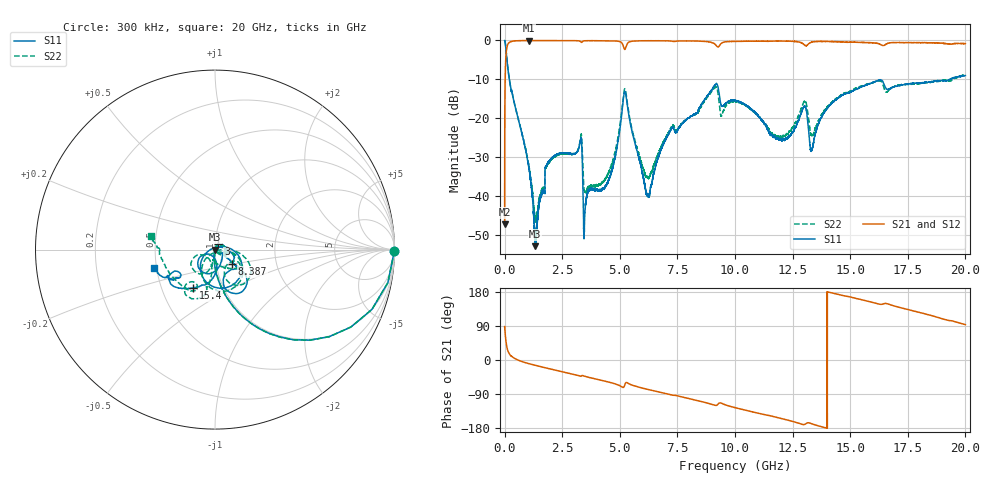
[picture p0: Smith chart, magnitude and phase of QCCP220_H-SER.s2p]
!{QCCP220}
!Johanson Technology Inc.
!www.johansontechnology.com
!Test Board Conditions:
!Substrate Type  RO4350B
!Substrate Thickness  20 mil
!Substrate Dk  3.66
!TL Type: GCPW
!TL Trace Width  36 mil
!TL Gap  12 mil
!Electrode orientation  Horizontal
!DUT TOPOLOGY	SERIES
!Mounting Pad LxW  26x36 mil
! Created Sat Jan  9 18:34:06 2021
# hz S ma R 50
! 2 Port Network Data from SP1.SP block
! freq  magS11  angS11  magS21  angS21  magS12  angS12  magS22  angS22
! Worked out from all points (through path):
!   20001 points, 300 kHz to 20 GHz, reference 50 ohm
!   highest |S21| = -0.02 dB at 1.049 GHz (marker M1); lowest = -47.3 dB at 300 kHz (marker M2)
!   group delay of S21, straight-line fit = 37.2 ps
!   lowest |S11| = -52.9 dB at 1.332 GHz (marker M3), VSWR 1.00, Z = 49.8 - j0.0174 ohm
!   |S11| at or under -10 dB: 205.2 MHz to 19.33 GHz (19.13 GHz wide, 196 % of centre)
!   |S22| runs from -46.7 to 0.0 dB; largest |S21 - S12| = 0.017
!   S11 on the Smith chart (normalised r, x): 300 kHz: open; 3 GHz: 1.04, +0.06; 8.387 GHz: 1.20, -0.19; 15.4 GHz: 0.72, -0.33; 20 GHz: 0.48, -0.11
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300000  0.9987 -0.5  0.0043 88.1  0.004282 89.0  1 -0.5
1.433e8  0.4341 -65.5  0.897 24.3  0.8978 24.2  0.4364 -65.4
1.0493e9  0.0236 -103.0  0.9981 -9.5  0.9976 -9.5  0.0249 -91.0
1.3323e9  0.002264 -175.6  0.9957 -14.1  0.9969 -14.0  0.005051 -31.8
1.8503e9  0.02568 65.8  0.9964 -21.7  0.9957 -21.7  0.02498 71.1
3.0003e9  0.03501 57.8  0.9935 -37.7  0.9938 -37.7  0.03477 46.3
3.3343e9  0.05381 -7.8  0.9443 -42.2  0.9445 -42.2  0.06104 -14.7
3.5003e9  0.0074 63.4  0.9906 -43.3  0.9903 -43.4  0.01128 -6.4
4.3843e9  0.01338 63.6  0.9914 -56.3  0.991 -56.2  0.01674 -7.8
5.2263e9  0.2214 -74.9  0.7677 -64.0  0.7664 -63.9  0.2388 -75.8
6.1913e9  0.01056 118.7  0.9907 -77.2  0.9924 -77.2  0.01761 -82.9
6.6673e9  0.03101 25.4  0.9919 -84.0  0.9905 -83.9  0.03491 -23.1
8.3873e9  0.1243 -39.5  0.9823 -107.4  0.9819 -107.4  0.1163 -4.2
9.1523e9  0.2725 -52.2  0.8825 -119.9  0.8861 -119.9  0.249 -42.8
9.4273e9  0.143 -61.9  0.9266 -114.4  0.9307 -114.4  0.1096 -41.6
1.00003e10  0.1688 -38.4  0.9726 -125.7  0.9718 -125.7  0.1647 -35.0
1.19673e10  0.05384 -28.8  0.9821 -153.7  0.9837 -153.7  0.0585 -98.2
1.30163e10  0.1426 -116.1  0.8725 -170.2  0.874 -170.2  0.1649 -130.5
1.33343e10  0.03929 -111.8  0.9518 -168.3  0.9527 -168.3  0.0606 -135.4
1.53963e10  0.2456 -119.6  0.9441 160.5  0.9494 160.2  0.2537 -102.5
1.66673e10  0.2353 -144.2  0.9262 147.2  0.9191 147.2  0.2277 -115.8
2e10  0.3543 -163.0  0.9109 93.2  0.8995 93.1  0.3667 168.0
